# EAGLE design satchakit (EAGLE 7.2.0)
CNAME: RDUINO V4; CREVISION: 4; DESIGNER: RODNEYD
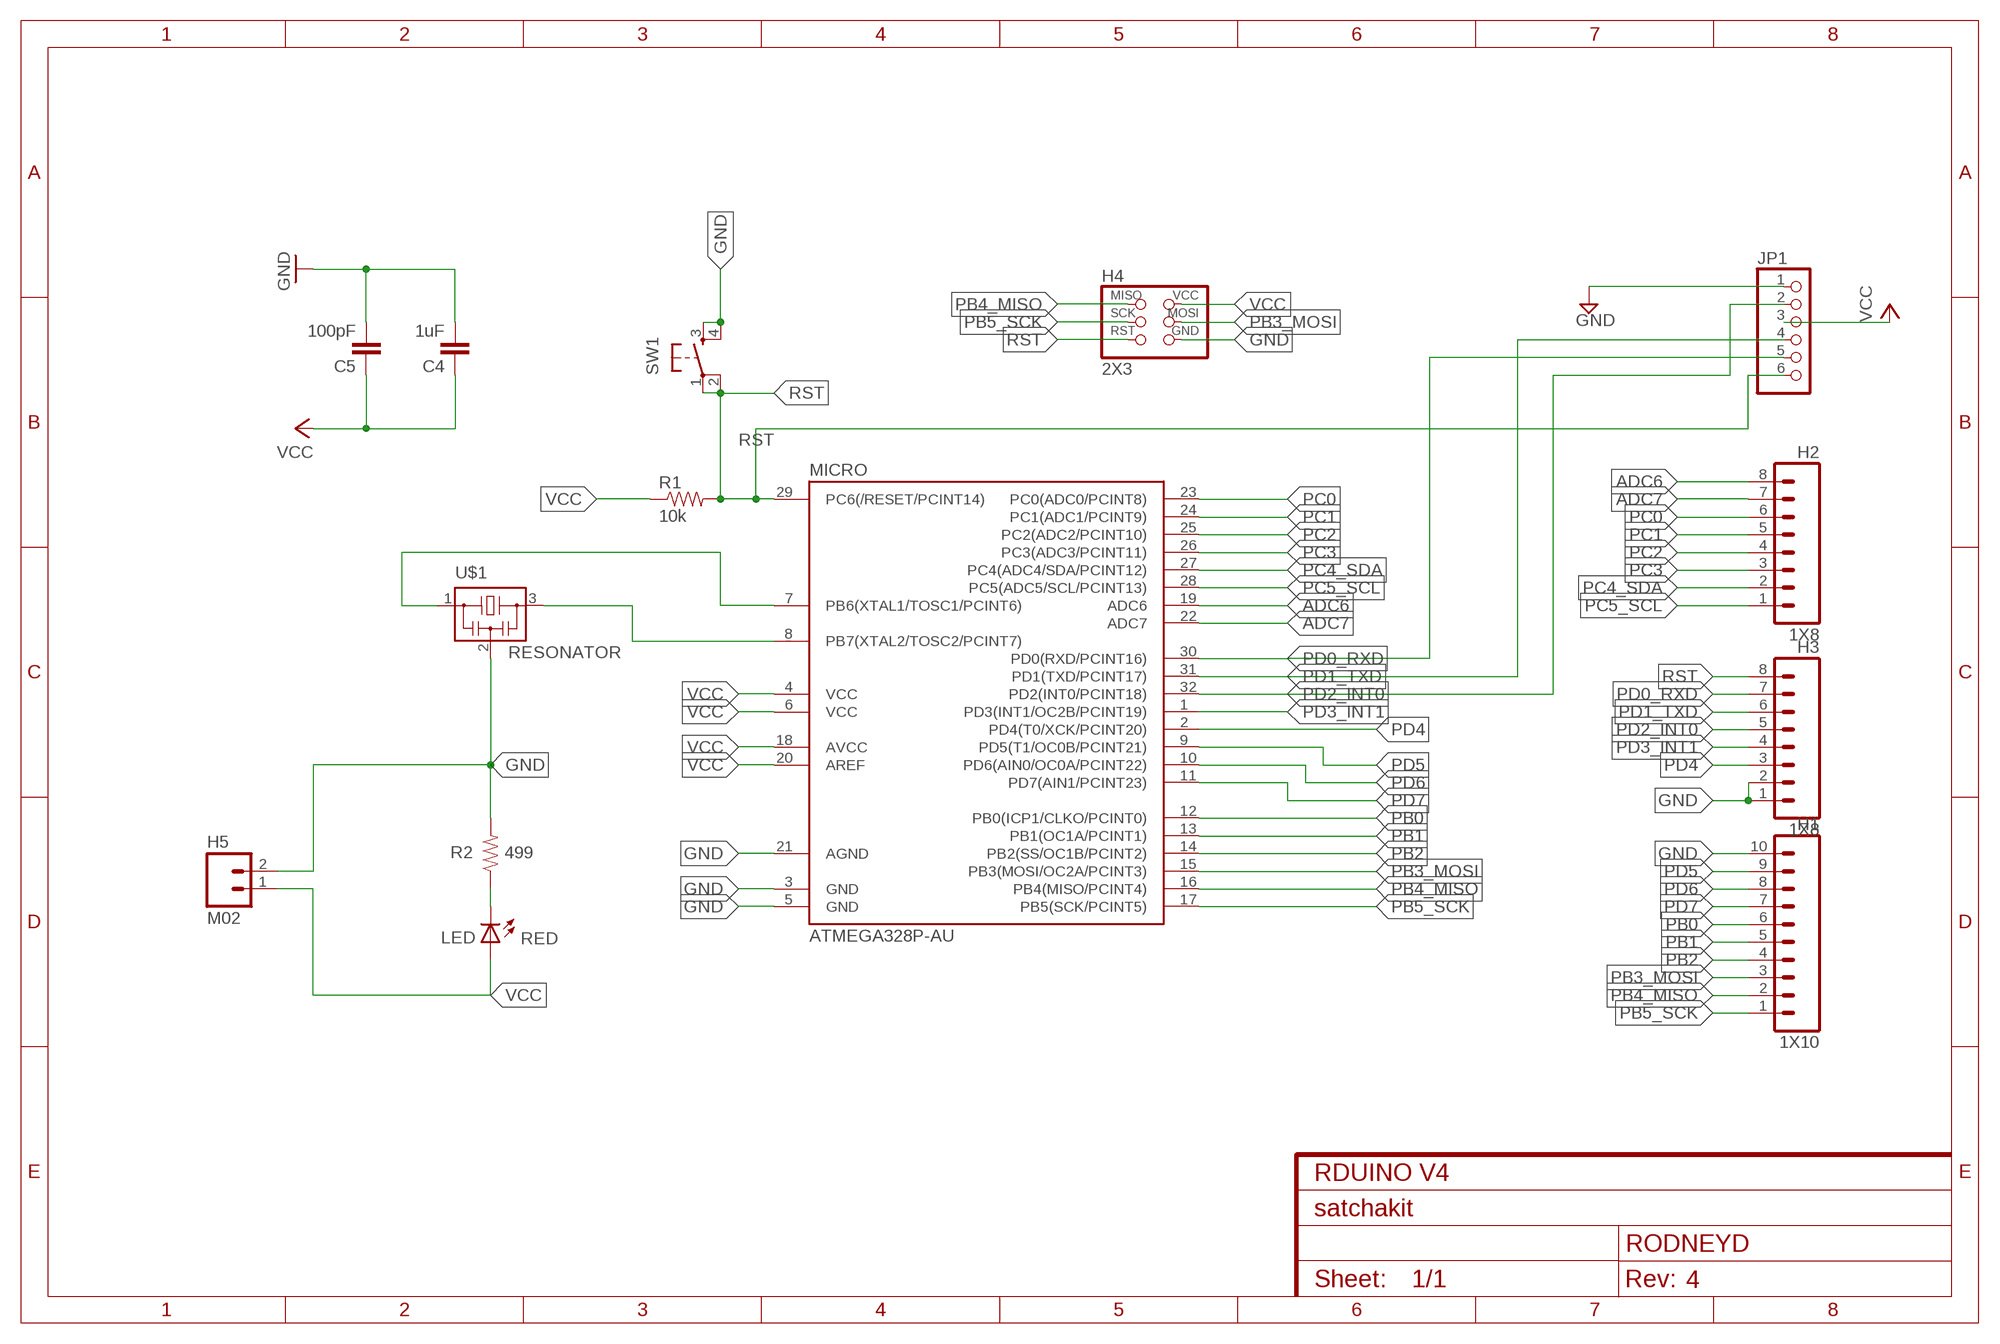
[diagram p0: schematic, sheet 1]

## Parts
C4  1uF  CAP1206  [1206]
C5  100pF  CAP1206  [1206]
H1  1X10  M101X10_SMD_STRAIGHT_ALT  [1X10_SMD_STRAIGHT_ALT]
H2  1X8  M081X08_SMD_STRAIGHT_ALT  [1X08_SMD_STRAIGHT_ALT]
H3  1X8  M081X08_SMD_STRAIGHT_ALT  [1X08_SMD_STRAIGHT_ALT]
H4  2X3  AVRISPSMD  [2X03SMD]
H5  M02  [1X02_SMD_FLAT_PADS]
JP1  PINHD-1X6  [1X06]
LED  RED  LED1206  [1206]
MICRO  ATMEGA328P-AU  ATMEGA48/88/168-AU  [TQFP32-08]
R1  10k  RESISTOR1206  [1206]
R2  499  RESISTOR1206  [1206]
SW1  6MM_SWITCH6MM_SWITCH  [6MM_SWITCH]
U$1  RESONATOR  [EFOBM]

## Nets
ADC6: H2.8 MICRO.19(ADC6)
ADC7: H2.7 MICRO.22(ADC7)
GND: C4.2 C5.2 H1.10 H3.1 H3.2 H4.6(GND) H5.2 JP1.1 MICRO.3(GND) MICRO.5(GND) MICRO.21(AGND) R2.2 SW1.3(S) SW1.4(S1) U$1.2
N$2: MICRO.8(PB7(XTAL2/TOSC2/PCINT7)) U$1.3
N$9: MICRO.7(PB6(XTAL1/TOSC1/PCINT6)) U$1.1
N$26: LED.2(C) R2.1
PB0: H1.6 MICRO.12(PB0(ICP1/CLKO/PCINT0))
PB1: H1.5 MICRO.13(PB1(OC1A/PCINT1))
PB2: H1.4 MICRO.14(PB2(SS/OC1B/PCINT2))
PB3_MOSI: H1.3 H4.4(MOSI) MICRO.15(PB3(MOSI/OC2A/PCINT3))
PB4_MISO: H1.2 H4.1(MISO) MICRO.16(PB4(MISO/PCINT4))
PB5_SCK: H1.1 H4.3(SCK) MICRO.17(PB5(SCK/PCINT5))
PC0: H2.6 MICRO.23(PC0(ADC0/PCINT8))
PC1: H2.5 MICRO.24(PC1(ADC1/PCINT9))
PC2: H2.4 MICRO.25(PC2(ADC2/PCINT10))
PC3: H2.3 MICRO.26(PC3(ADC3/PCINT11))
PC4_SDA: H2.2 MICRO.27(PC4(ADC4/SDA/PCINT12))
PC5_SCL: H2.1 MICRO.28(PC5(ADC5/SCL/PCINT13))
PD0_RXD: H3.7 JP1.5 MICRO.30(PD0(RXD/PCINT16))
PD1_TXD: H3.6 JP1.4 MICRO.31(PD1(TXD/PCINT17))
PD2_INT0: H3.5 JP1.2 MICRO.32(PD2(INT0/PCINT18))
PD3_INT1: H3.4 MICRO.1(PD3(INT1/OC2B/PCINT19))
PD4: H3.3 MICRO.2(PD4(T0/XCK/PCINT20))
PD5: H1.9 MICRO.9(PD5(T1/OC0B/PCINT21))
PD6: H1.8 MICRO.10(PD6(AIN0/OC0A/PCINT22))
PD7: H1.7 MICRO.11(PD7(AIN1/PCINT23))
RST: H3.8 H4.5(RST) JP1.6 MICRO.29(PC6(/RESET/PCINT14)) R1.2 SW1.1(P) SW1.2(P1)
VCC: C4.1 C5.1 H4.2(VCC) H5.1 JP1.3 LED.1(A) MICRO.4(VCC) MICRO.6(VCC) MICRO.18(AVCC) MICRO.20(AREF) R1.1

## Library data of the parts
C4 C5 = 01_SparkFun:CAP: Capacitor
H1 = Working:M10
H2 H3 = Working:M08
H4 = fab:AVRISP
H5 = Working:M02
JP1 = pinhead:PINHD-1X6: PIN HEADER
LED = 01_FAB_Hello:LED
MICRO = atmega8:ATMEGA48/88/168
R1 R2 = 01_SparkFun:RESISTOR: Resistor
SW1 = 01_FAB_Hello:6MM_SWITCH: OMRON SWITCH
U$1 = fab:RESONATOR

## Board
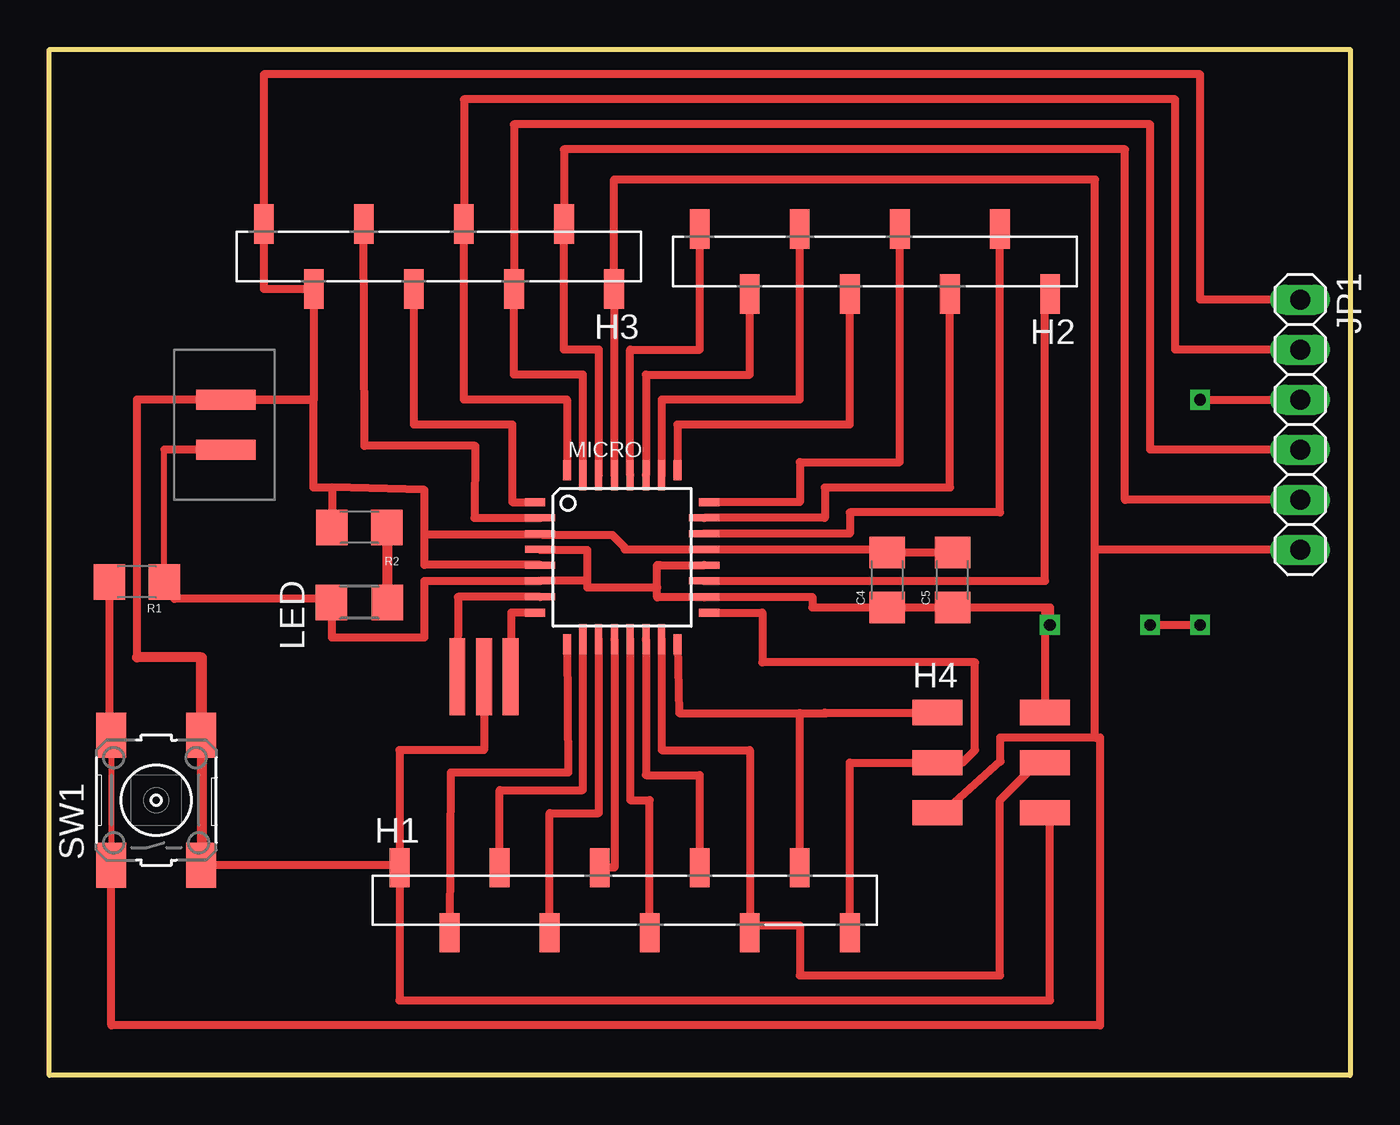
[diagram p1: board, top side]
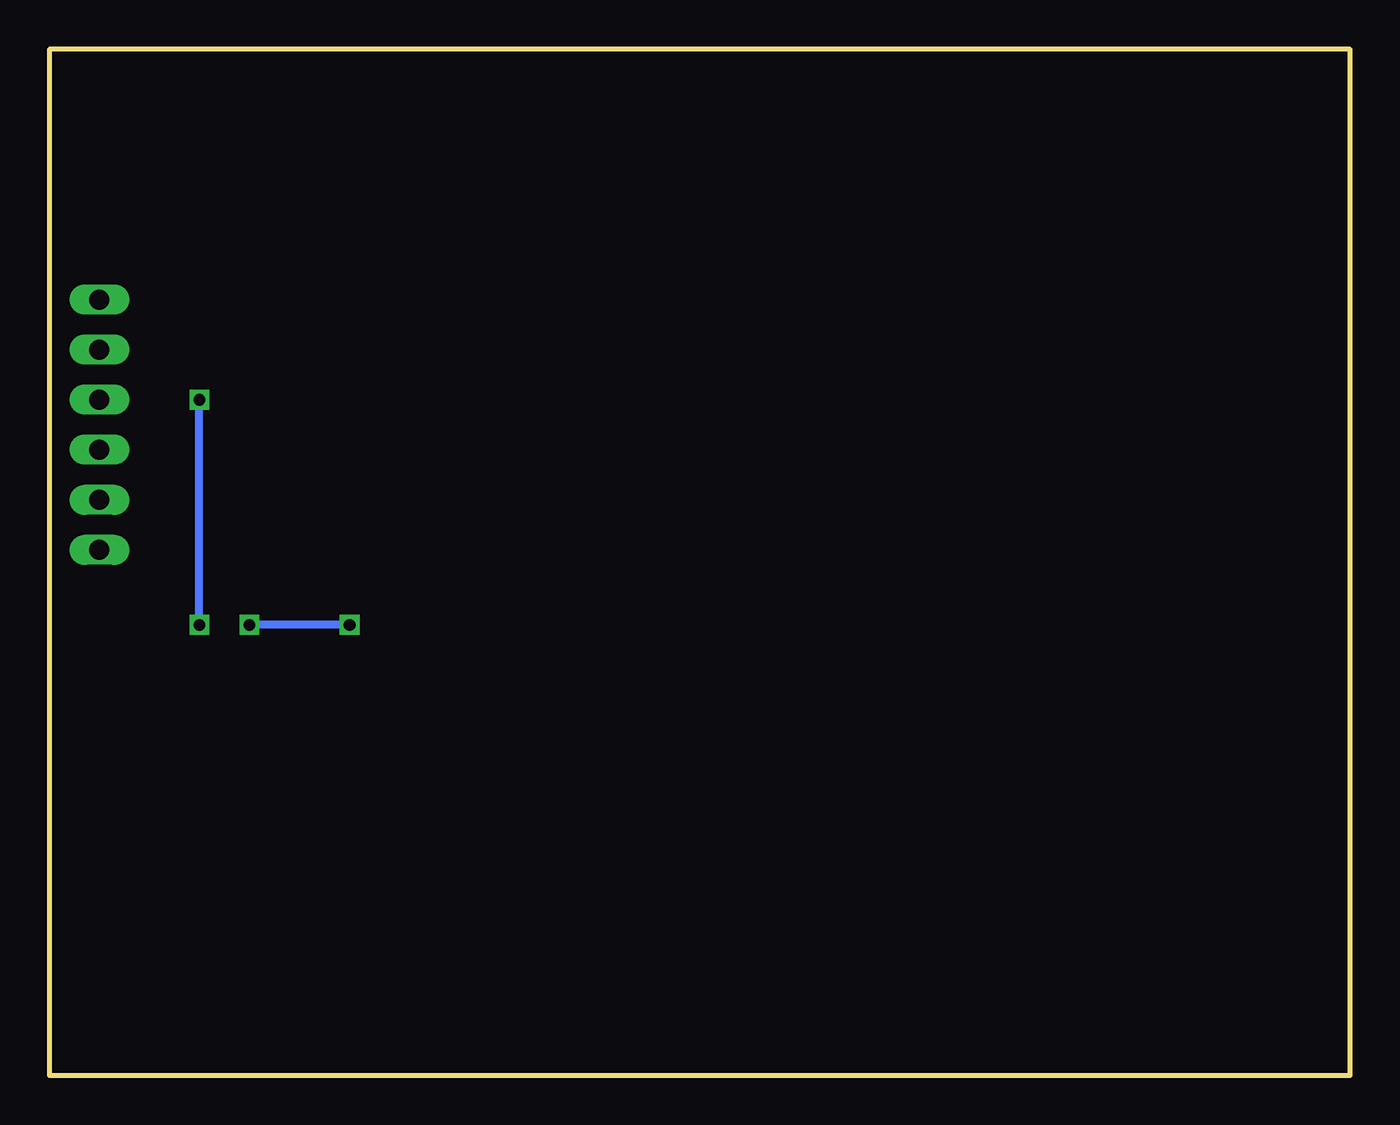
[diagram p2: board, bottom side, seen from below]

Size 66.04 x 52.07 mm. Coordinates in mm from the lower left corner, seen from the top.
Outline: 0,0 0,52.07 66.04,52.07 66.04,0 0,0
Copper layers (1*16): Top 0.035mm / dielectric 1.5mm / Bottom 0.035mm
Design rules "default *": minimum track width 12mil, minimum drill 24mil, track to track 12mil, track to pad 12mil, pad to pad 8mil, via to via 8mil, smd to smd 8mil, copper to edge 40mil, drill to drill 8mil, minimum pad ring 10mil, minimum via ring 8mil, stop-mask expansion 4mil, vias tented up to drill 0mil, thermal gap 10mil

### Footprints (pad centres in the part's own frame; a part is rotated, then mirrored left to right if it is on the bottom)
1206 = smd 1.6 x 1.8: 1 -1.4,0; 2 1.4,0
1X10_SMD_STRAIGHT_ALT = smd 1 x 2: 1 -1.27,-0.38; 2 -3.81,2.92; 3 -6.35,-0.38; 4 -8.89,2.92; 5 -11.43,-0.38; 6 -13.97,2.92; 7 -16.51,-0.38; 8 -19.05,2.92; 9 -21.59,-0.38; 10 -24.13,2.92
1X08_SMD_STRAIGHT_ALT = smd 1 x 2: 1 -1.27,-0.38; 2 -3.81,2.92; 3 -6.35,-0.38; 4 -8.89,2.92; 5 -11.43,-0.38; 6 -13.97,2.92; 7 -16.51,-0.38; 8 -19.05,2.92
2X03SMD = smd 2.54 x 1.27: 1 -2.54,2.54; 2 2.92,2.54; 3 -2.54,0; 4 2.92,0; 5 -2.54,-2.54; 6 2.92,-2.54
1X02_SMD_FLAT_PADS = smd 1 x 3: 1 2.54,1.19; 2 5.08,1.19
1X06 = drill 1.016 long: 1 -6.35,0; 2 -3.81,0; 3 -1.27,0; 4 1.27,0; 5 3.81,0; 6 6.35,0
1206' = smd 1.6 x 1.803: 1 -1.422,0; 2 1.422,0
TQFP32-08 = smd 1.016 x 0.406: 1 -4.42,2.8; 8 -4.42,-2.8; 17 4.42,-2.8; 24 4.42,2.8 | smd 1.524 x 0.356: 2 -4.166,2; 3 -4.166,1.2; 4 -4.166,0.4; 5 -4.166,-0.4; 6 -4.166,-1.2; 7 -4.166,-2; 18 4.166,-2; 19 4.166,-1.2; 20 4.166,-0.4; 21 4.166,0.4; 22 4.166,1.2; 23 4.166,2 | smd 0.406 x 1.016: 9 -2.8,-4.42; 16 2.8,-4.42; 25 2.8,4.42; 32 -2.8,4.42 | smd 0.356 x 1.524: 10 -2,-4.166; 11 -1.2,-4.166; 12 -0.4,-4.166; 13 0.4,-4.166; 14 1.2,-4.166; 15 2,-4.166; 26 2,4.166; 27 1.2,4.166; 28 0.4,4.166; 29 -0.4,4.166; 30 -1.2,4.166; 31 -2,4.166
6MM_SWITCH = smd 2.286 x 1.524: 1 -3.302,2.286; 2 3.302,2.286; 3 -3.302,-2.286; 4 3.302,-2.286
EFOBM = smd 0.8 x 3.9: 1 -1.35,0; 2 0,0; 3 1.35,0

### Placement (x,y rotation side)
C4  42.55,25.15 90 top
C5  45.85,25.15 90 top
H1  41.91,7.62 0 top
H2  31.75,42.58 180 top
H3  9.62,42.83 180 top
H4  47.62,15.88 0 top
H5  10.16,29.21 90 top
JP1  63.5,33.02 270 top
LED  RED  [1206']  15.75,24 0 top
MICRO  29.08,26.29 0 top
R1  4.45,25.04 180 top
R2  15.75,27.81 180 top
SW1  5.44,13.97 90 top
U$1  22.07,20.22 0 top

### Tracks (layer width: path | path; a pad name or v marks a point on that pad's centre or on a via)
ADC6
  Top 0.406: MICRO.19 50.55,25.09 50.55,39.66 H2.8
ADC7
  Top 0.406: MICRO.22 40.64,27.49 40.64,28.57 48.26,28.57 H2.7
GND
  Top 0.305: SW1.4 SW1.3 | MICRO.5 24.92,25.91 | MICRO.21 | MICRO.3 25.04,27.43 | 50.27,13.31 H4.6 | H1.10 17.68,10.46 17.78,10.46
  Top 0.406: 24.92,25.91 19.05,25.91 19.05,27.43 | 19.05,27.43 19.05,29.72 14.35,29.84 | 14.35,29.84 R2.2 | 19.05,27.43 25.04,27.43 28.57,27.43 29.21,26.8 29.21,26.69 MICRO.21 42.55,26.69 C4.2 C5.2 | 4.45,21.21 4.45,34.29 H5.2 | 14.35,27.94 R2.2 | U$1.2 22.07,16.51 17.78,16.51 17.78,10.67 | H5.2 13.43,34.29 H3.2 10.89,39.91 H3.1 10.89,50.8 58.42,50.8 58.42,39.37 JP1.1 | H5.2 13.4,34.29 13.4,29.84 14.35,29.84 | 17.78,10.67 SW1.3 | 17.78,10.67 H1.10 17.78,10.46 17.78,3.81 50.8,3.81 50.8,13.34 H4.6
  Top 0.508: SW1.4 7.72,21.21 | 7.72,21.21 4.45,21.21 | 7.72,21.21 7.75,21.21 7.75,10.54 | R2.2
N$2
  Top 0.406: MICRO.8 23.45,23.49 U$1.3
N$9
  Top 0.406: MICRO.7 20.75,24.29 U$1.1
N$26
  Top 0.508: R2.1 17.15,24 LED.2
PB0
  Top 0.305: MICRO.12 28.7,22.12
  Top 0.406: MICRO.12 28.68,10.54 H1.6
PB1
  Top 0.406: MICRO.13 29.48,13.97 30.48,13.97 H1.5
PB2
  Top 0.406: MICRO.14 30.28,15.24 33.02,15.24 H1.4
PB3_MOSI
  Top 0.305: 50.27,15.75 H4.4
  Top 0.406: MICRO.15 31.08,16.51 35.56,16.51 H1.3 35.56,7.62 38.1,7.62 38.1,5.08 48.26,5.08 48.26,13.97 50.16,15.88 H4.4
PB4_MISO
  Top 0.305: MICRO.16 | 45.09,18.19 H4.1
  Top 0.406: MICRO.16 31.98,18.38 38.1,18.38 | 38.1,18.38 39.47,18.38 39.37,18.41 H4.1 | H1.2 38.1,18.38
PB5_SCK
  Top 0.305: 45.09,16.05 H4.3
  Top 0.406: MICRO.17 36.2,23.49 36.2,20.95 46.99,20.95 46.99,16.51 46.35,15.88 H4.3 40.64,15.88 H1.1
PC0
  Top 0.406: MICRO.23 39.37,28.29 39.37,29.84 45.72,29.84 H2.6
PC1
  Top 0.406: MICRO.24 38.1,29.09 38.1,31.11 43.18,31.11 H2.5
PC2
  Top 0.406: MICRO.25 31.88,33.02 40.64,33.02 H2.4
PC3
  Top 0.406: MICRO.26 31.08,34.29 38.1,34.29 H2.3
PC4_SDA
  Top 0.406: MICRO.27 30.28,35.56 35.56,35.56 H2.2
PC5_SCL
  Top 0.406: MICRO.28 29.48,36.83 33.02,36.83 H2.1
PD0_RXD
  Top 0.406: MICRO.30 27.88,36.83 26.13,36.83 H3.7 26.13,46.99 54.61,46.99 54.61,29.21 JP1.5
PD1_TXD
  Top 0.406: MICRO.31 27.08,35.56 23.59,35.56 H3.6 23.59,48.26 55.88,48.26 55.88,31.75 JP1.4
PD2_INT0
  Top 0.406: MICRO.32 26.28,34.29 21.05,34.29 H3.5 21.05,49.53 57.15,49.53 57.15,36.83 JP1.2
PD3_INT1
  Top 0.406: MICRO.1 23.5,29.09 23.5,33.02 18.51,33.02 H3.4
PD4
  Top 0.406: MICRO.2 21.59,28.29 21.62,31.94 16,31.94 H3.3
PD5
  Top 0.406: MICRO.9 26.35,15.37 20.38,15.37 H1.9
PD6
  Top 0.406: MICRO.10 27.08,14.48 22.86,14.48 H1.8
PD7
  Top 0.406: MICRO.11 27.88,13.31 25.4,13.31 H1.7
RST
  Top 0.305: SW1.2 SW1.1 | MICRO.29 28.7,30.45 | 45.7,13.61 45.09,13.61 H4.5
  Top 0.406: 53.09,17.14 53.09,26.67 | 53.09,26.67 53.09,45.47 28.67,45.47 H3.8 28.68,39.91 MICRO.29 | R1.2 3.04,17.27 SW1.2 | 53.09,17.14 48.26,17.14 48.26,15.94 48.29,15.94 45.7,13.61 | 53.09,17.14 53.34,17.14 53.34,2.54 3.15,2.54 SW1.1 | JP1.6 53.09,26.67
VCC  (via drill 0.6)
  Top 0.305: R1.1 5.84,31.75 | MICRO.18 33.25,24.26 | 30.86,25.91 30.99,25.91 30.99,25.89 | MICRO.4 24.92,26.67 | MICRO.6 24.79,25.15 | 50.27,18.49 H4.2 | LED.1 14.33,24.18 14.35,24
  Top 0.406: 33.25,24.26 30.86,24.26 30.86,24.77 | 30.86,24.77 30.86,25.91 | 30.99,25.89 MICRO.20 | 14.35,24 14.35,22.22 19.05,22.22 19.05,25.09 MICRO.6 27.3,25.09 | 24.92,26.67 27.3,26.67 27.3,25.09 | 27.3,25.09 27.3,24.77 30.86,24.77 | MICRO.18 38.73,24.29 38.73,23.75 C4.1 C5.1 50.55,23.75 | H5.1 5.84,31.75 | 50.55,23.75 H4.2 | 50.55,23.75 50.8,23.75 v50.8,22.86 | v55.88,22.86 v58.42,22.86 | v58.42,34.29 JP1.3 | 14.33,24.18 6.35,24.18 6.35,25.4 5.84,25.4 R1.1
  Bottom 0.406: v50.8,22.86 v55.88,22.86 | v58.42,22.86 v58.42,34.29

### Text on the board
tDocu: RDuino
